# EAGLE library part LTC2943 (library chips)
Multicell Battery Gas Gauge with Temperature, Voltage and Current Measurement
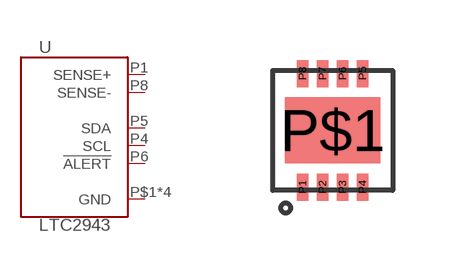
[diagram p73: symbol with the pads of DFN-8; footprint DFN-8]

Designator prefix U

## LTC2943 (DIGIKEY: LTC2943IDD#PBF-ND)  [DFN-8]
P1  SENSE+  oc
P2  GND  oc
P3  GND  oc
P4  SCL  oc
P5  SDA  oc
P6  !ALERT  oc
P7  GND  oc
P8  SENSE-  oc
P$1  GND  oc

## Footprint DFN-8 (pad centres in mm)
smd 0.28 x 0.675: P1 -0.75,-1.42; P2 -0.25,-1.42; P3 0.25,-1.42; P4 0.75,-1.42; P5 0.75,1.42; P6 0.25,1.42; P7 -0.25,1.42; P8 -0.75,1.42
smd 2.38 x 1.65: P$1 0,0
